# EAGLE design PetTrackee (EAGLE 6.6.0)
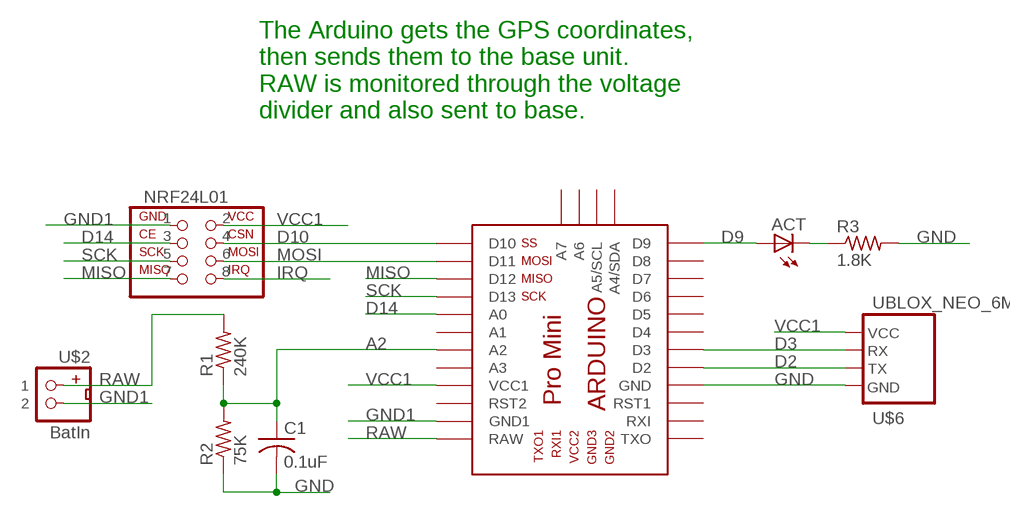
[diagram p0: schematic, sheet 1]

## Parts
ACT  LED3MM  [LED3MM]
C1  0.1uF  C-US025-025X050  [C025-025X050]
NRF24L01  NRF24L01+  [NRF24L01+]
R1  240K  R-US_0207/10  [0207/10]
R2  75K  R-US_0207/10  [0207/10]
R3  1.8K  R-US_0207/10  [0207/10]
U$1  PRO_MINI  [PRO_MINI]
U$2  BatIn  JST2.0  [JST2.0]
U$6  UBLOX_NEO_6M  [UBLOX_NEO_6M]

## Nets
A2: C1.1 R1.1 R2.2 U$1.A2
D2: U$1.D2 U$6.TX
D3: U$1.D3 U$6.RX
D9: ACT.A U$1.D9
D10: NRF24L01.4 U$1.D10
D14: NRF24L01.3 U$1.A0
GND [power]: C1.2 R2.1 R3.2 U$1.GND U$6.GND
GND1 [power]: NRF24L01.1 U$1.GND1 U$2.2
IRQ: NRF24L01.8
MISO: NRF24L01.7 U$1.D12
MOSI: NRF24L01.6 U$1.D11
N$2: ACT.K(C) R3.1
RAW: R1.2 U$1.RAW U$2.1
SCK: NRF24L01.5 U$1.D13
VCC1: NRF24L01.2 U$1.VCC1 U$6.VCC
Unconnected: U$1.A1 U$1.A3 U$1.A4(A4/SDA) U$1.A5(A5/SCL) U$1.A6 U$1.A7 U$1.D4 U$1.D5 U$1.D6 U$1.D7 U$1.D8 U$1.RST1 U$1.RST2 U$1.RXI U$1.TXO

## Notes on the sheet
- The Arduino gets the GPS coordinates, 
  then sends them to the base unit.
  RAW is monitored through the voltage 
  divider and also sent to base.

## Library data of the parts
ACT = SparkFun:LED: LEDs
C1 = rcl:C-US: CAPACITOR, American symbol
NRF24L01 = MTS_Custom:NRF24L01+
R1-R3 = rcl:R-US_: RESISTOR, American symbol
U$1 = MTS_Custom:PRO_MINI
U$2 = MTS_Custom:JST2.0
U$6 = MTS_Custom:UBLOX_NEO_6M

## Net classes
0 default: width 0.305 mm
1 power: width 0.6 mm, clearance 0.3 mm

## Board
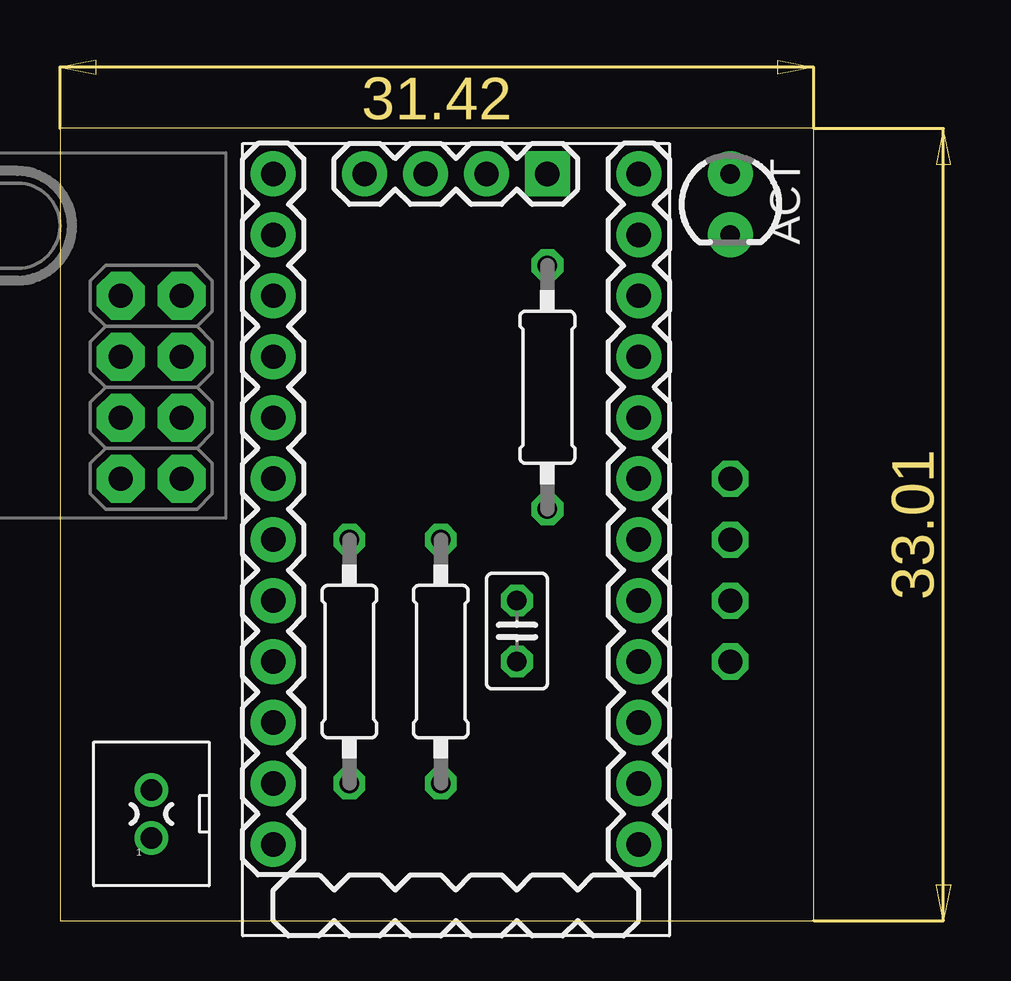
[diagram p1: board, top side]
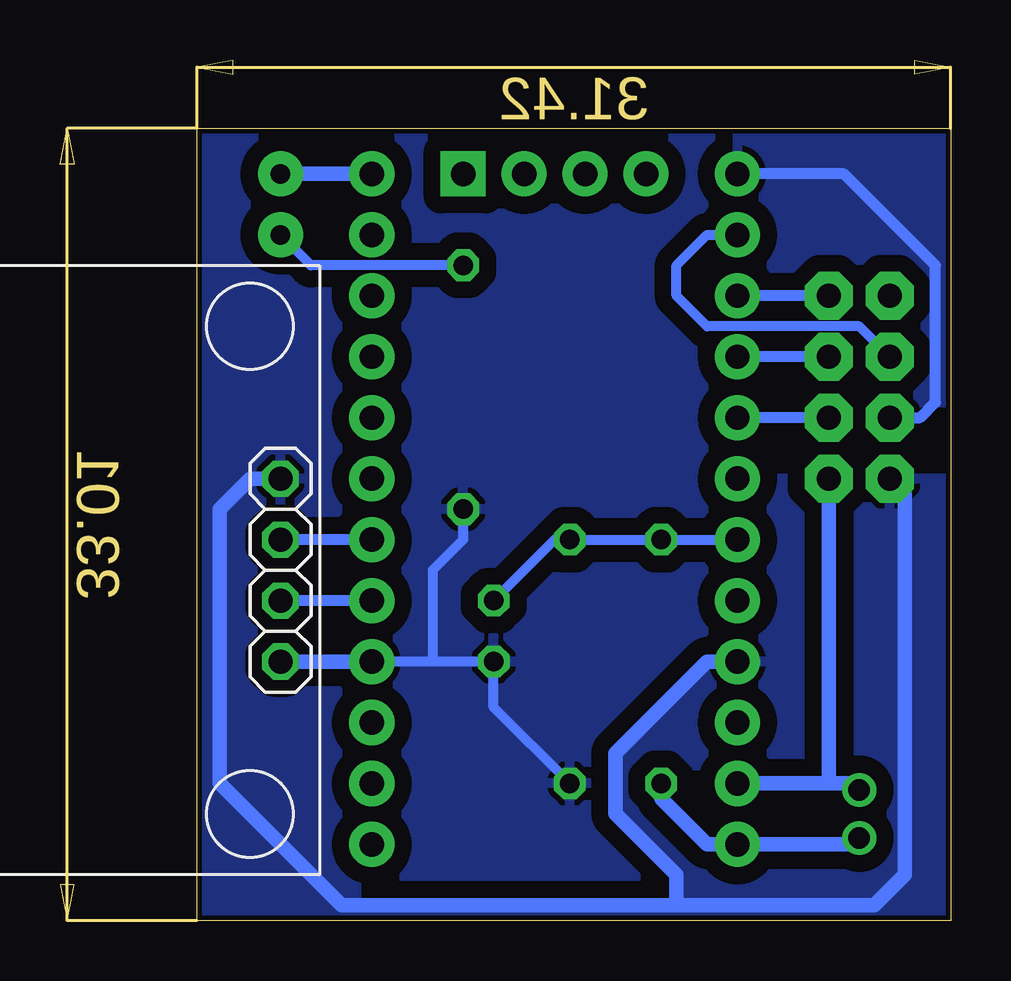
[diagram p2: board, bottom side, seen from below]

Size 37.13 x 35.86 mm. Coordinates in mm from the lower left corner, seen from the top.
Outline: 0,0 31.42,0 31.42,33.01 0,33.01 0,0
Copper layers (1*16): Top 0.035mm / dielectric 1.5mm / Bottom 0.035mm
Design rules "MTS *": minimum track width 20mil, minimum drill 12mil, track to track 28mil, track to pad 28mil, pad to pad 6mil, via to via 6mil, smd to smd 0mil, copper to edge 8mil, drill to drill 10mil, minimum pad ring 10mil, minimum via ring 10mil, stop-mask expansion 2mil, vias tented up to drill 25mil, thermal gap 10mil

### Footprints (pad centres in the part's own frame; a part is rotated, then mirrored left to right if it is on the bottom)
LED3MM = drill 0.813 pad 1.88: A -1.27,0; K 1.27,0
C025-025X050 = drill 0.813 octagon: 1 -1.27,0; 2 1.27,0
NRF24L01+ = drill 1 pad 2 octagon: 1 -5.08,-12.7; 2 -5.08,-10.16; 3 -2.54,-12.7; 4 -2.54,-10.16; 5 0,-12.7; 6 0,-10.16; 7 2.54,-12.7; 8 2.54,-10.16
0207/10 = drill 0.813 octagon: 1 -5.08,0; 2 5.08,0
PRO_MINI = drill 1.016 pad 1.88: A0 -5.08,-7.62; A1 -2.54,-7.62; A2 0,-7.62; A3 2.54,-7.62; A5 -15.24,1.27; A6 -15.24,-1.27; A7 -15.24,-3.81; D2 2.54,7.62; D3 0,7.62; D4 -2.54,7.62; D5 -5.08,7.62; D6 -7.62,7.62; D7 -10.16,7.62; D8 -12.7,7.62; D9 -15.24,7.62; D10 -15.24,-7.62; D11 -12.7,-7.62; D12 -10.16,-7.62; D13 -7.62,-7.62; GND 5.08,7.62; GND1 10.16,-7.62; RAW 12.7,-7.62; RST1 7.62,7.62; RST2 7.62,-7.62; RXI 10.16,7.62; TXO 12.7,7.62; VCC1 5.08,-7.62 | drill 1.016 pad 1.88 square: A4 -15.24,3.81
JST2.0 = drill 0.9 pad 1.016: 1 0,-1; 2 0,1
UBLOX_NEO_6M = drill 1 octagon: GND -16.51,3.81; RX -16.51,-1.27; TX -16.51,1.27; VCC -16.51,-3.81

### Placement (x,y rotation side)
ACT  27.94,29.84 270 top
C1  19.05,12.06 270 top
NRF24L01  -7.62,23.5 90 top
R1  12.06,10.79 270 top
R2  15.88,10.79 90 top
R3  20.32,22.23 270 top
U$1  16.51,15.88 270 top
U$2  3.81,4.45 0 top
U$6  44.45,14.61 180 bottom

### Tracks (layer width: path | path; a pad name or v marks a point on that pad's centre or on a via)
A2
  Bottom 0.406: C1.1 16.51,15.88 R2.2 R1.1 U$1.A2
D2
  Bottom 0.457: U$1.D2 U$6.TX
D3
  Bottom 0.457: U$1.D3 U$6.RX
D9
  Bottom 0.61: U$1.D9 ACT.A
D10
  Bottom 0.457: U$1.D10 4.45,31.11 0.64,27.3 0.64,21.59 1.27,20.95 NRF24L01.4
  pour Bottom: -1.27,21.59 -1.27,33.02 8.89,33.02 8.89,21.59
D14
  Bottom 0.457: NRF24L01.3 U$1.A0
GND
  Bottom 0.406: 21.59,10.79 C1.2 19.05,8.89 R2.1 | 21.59,10.79 U$1.GND | R3.2 20.32,15.88 21.59,14.61 21.59,10.79
  Bottom 0.6: U$1.GND U$6.GND
  pour Bottom: 8.89,33.02 24.13,33.02 24.13,1.27 12.7,1.27 12.7,2.54 13.97,3.81 13.97,7.62 8.89,12.7
GND1
  Bottom 0.61: U$1.GND1 5.08,5.71 | 5.08,5.71 4.08,5.71 U$2.2 | NRF24L01.1 5.08,5.71
MISO
  Bottom 0.457: NRF24L01.7 U$1.D12
MOSI
  Bottom 0.406: NRF24L01.6 3.81,24.77 10.16,24.77 11.43,26.04 11.43,27.3 10.16,28.57 U$1.D11
N$2
  Bottom 0.406: R3.1 26.67,27.3 ACT.K
RAW
  Bottom 0.61: R1.2 12.06,5.08 10.16,3.17 U$1.RAW 4.08,3.17 U$2.1
SCK
  Bottom 0.457: NRF24L01.5 U$1.D13
VCC1
  Bottom 0.61: U$1.VCC1 10.16,10.79 13.97,6.99 13.97,4.45 11.43,1.91 11.43,0.64 | NRF24L01.2 1.91,17.78 1.91,1.91 3.17,0.64 11.43,0.64 | U$6.VCC 29.21,18.41 30.48,17.14 30.48,5.71 25.4,0.64 11.43,0.64
  pour Bottom: -1.27,18.41 8.89,18.41 8.89,11.43 9.53,10.79 10.16,10.79 13.97,6.99 13.97,4.45 11.43,1.91 11.43,0.64 24.77,0.64 24.77,33.02 32.38,33.02 32.38,0 31.75,-0.64 -0.64,-0.64 -1.27,0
